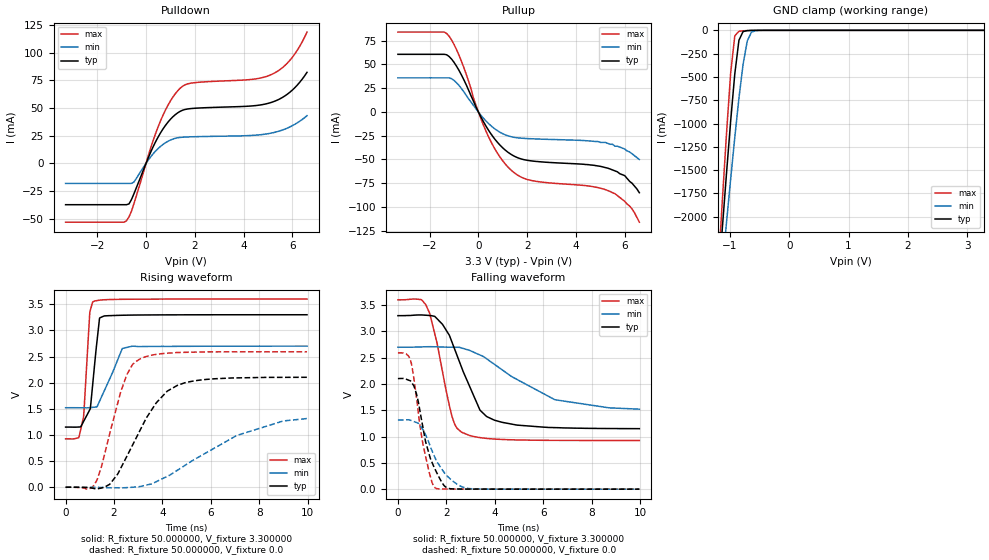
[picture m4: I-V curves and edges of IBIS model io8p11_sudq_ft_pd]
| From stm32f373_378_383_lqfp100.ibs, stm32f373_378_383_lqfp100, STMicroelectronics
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|   Model io8p11_sudq_ft_pd
[Model]  io8p11_sudq_ft_pd
Model_type I/O
Polarity   Non-Inverting
Enable   Active-Low
Vinl =   0.990000V
Vinh =   2.310000V
Vmeas =  1.650000V
Cref =   30.000000pF
Rref =   100.000000M
Vref =   0.0V
C_comp   1.970900pF   1.892300pF   2.063200pF
[Temperature Range]   25.000000   0.125000k   -40.000000
[Pullup Reference]   3.300000V   2.700000V   3.600000V
[Pulldown Reference]   0.0V   0.0V   0.0V
[POWER Clamp Reference]   3.300000V   2.700000V   3.600000V
[GND Clamp Reference]   0.0V   0.0V   0.0V
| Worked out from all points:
|   slope of the pulldown table from 0 to 0.495 V, typ, clamps not added: 20.9 ohm
|   slope of the pullup table from 0 to 0.495 V, typ, clamps not added: 22.2 ohm
|   GND clamp passes 1 mA (typ) near -0.64 V on its own axis
|   rising waveform, R_fixture 50.000000, V_fixture 3.300000: 20-80 % time 277ps typ, 663ps min, 203ps max; typ from 1.15 V to 3.3 V
|   rising waveform, R_fixture 50.000000, V_fixture 0.0: 20-80 % time 1.54ns typ, 3.09ns min, 916ps max; typ from 0 V to 2.1 V
|   falling waveform, R_fixture 50.000000, V_fixture 3.300000: 20-80 % time 1.14ns typ, 2.54ns min, 732ps max; typ from 3.3 V to 1.15 V
|   falling waveform, R_fixture 50.000000, V_fixture 0.0: 20-80 % time 659ps typ, 874ps min, 527ps max; typ from 2.1 V to 0 V
[Pulldown]
|Voltage   I(typ)   I(min)   I(max)
-3.3V     -37.45mA   -18.2mA    -53.24mA
-800mV    -37.45mA   -18.2mA    -51.9mA
-700mV    -36.7mA    -18.2mA    -48.48mA
-500mV    -27.71mA   -17.01mA   -36.66mA
200mV     10.57mA    6.084mA    14.57mA
500mV     23.91mA    13.38mA    33.24mA
900mV     37.17mA    19.88mA    52.48mA
1.3V      45.55mA    23.01mA    65.5mA
1.8V      49.29mA    23.83mA    72.18mA
5.1V      54.68mA    27.07mA    79.72mA
5.9V      64.2mA     32.82mA    93.01mA
6.6V      82.13mA    42.97mA    118.5mA
[Pullup]
|Voltage   I(typ)   I(min)   I(max)
-3.3V     60.68mA    35.92mA    84.08mA
-1.4V     60.68mA    35.92mA    84.08mA
-1.2V     58.37mA    35.92mA    79.66mA
-700mV    39.18mA    24.86mA    53.69mA
0V        0A         0A         0A
400mV     -18.61mA   -11.78mA   -25.23mA
900mV     -35.28mA   -21.55mA   -48mA
1.5V      -46.91mA   -26.86mA   -64.58mA
2.2V      -51.57mA   -28.22mA   -72.25mA
5.3V      -59.1mA    -33mA      -82.6mA
6.2V      -73mA      -42mA      -99mA
6.6V      -85mA      -50mA      -116mA
[GND_clamp]
|Voltage   I(typ)   I(min)   I(max)
-3.3V     -9.525A    -9.501A    -9.513A
-1.2V     -2.719A    -3.023A    -2.568A
-1.13V    -2.122A    -2.541A    -1.826A
-1.06V    -1.537A    -2.065A    -1.111A
-990mV    -975.7mA   -1.599A    -462mA
-920mV    -467.5mA   -1.149A    -59.02mA
-850mV    -106.6mA   -727.3mA   -10.13mA
-780mV    -13.08mA   -365.4mA   -5.271mA
-710mV    -3.06mA    -114.8mA   -2.651mA
-640mV    -957.2uA   -20.17mA   -921.6uA
-570mV    -212.9uA   -3.969mA   -172uA
3.28V     83.81uA    63.75uA    93.54uA
[POWER_clamp]
|Voltage   I(typ)   I(min)   I(max)
-3.28V    0A         0A         0A
0V        0A         0A         0A
[Ramp]
| variable   typ   min   max
dV/dt_r  1.26120/1.54122n   0.74130/3.11733n   1.55376/0.91453n
dV/dt_f  1.28796/1.14240n   0.68838/2.56706n   1.60431/0.73092n
R_load = 50.000000
[Rising Waveform]
R_fixture= 50.000000
V_fixture= 3.300000
V_fixture_min= 2.700000
V_fixture_max= 3.600000
|time   V(typ)   V(min)   V(max)
0s        1.15V      1.521V     925.1mV
540.5ps   1.152V     1.52V      945.8mV
740.7ps   1.256V     1.519V     1.344V
1.001ns   1.484V     1.523V     3.353V
1.121ns   1.976V     1.528V     3.546V
1.401ns   3.231V     1.644V     3.577V
1.602ns   3.276V     1.848V     3.585V
2.342ns   3.289V     2.654V     3.594V
2.763ns   3.292V     2.698V     3.595V
9.97ns    3.299V     2.699V     3.599V
[Rising Waveform]
R_fixture= 50.000000
V_fixture= 0.0
V_fixture_min= 0.0
V_fixture_max= 0.0
|time   V(typ)   V(min)   V(max)
0s        -11.46uV   -27.3uV    -6.454uV
1.181ns   -24.48mV   -1.038mV   43.68mV
1.481ns   -14.37mV   -4.325mV   396.7mV
1.822ns   56.8mV     -9.542mV   1.023V
2.523ns   585.5mV    -6.904mV   2.147V
3.043ns   1.06V      10.75mV    2.445V
3.744ns   1.614V     106.7mV    2.541V
4.905ns   1.995V     410.6mV    2.58V
7.067ns   2.091V     989.9mV    2.59V
9.97ns    2.103V     1.315V     2.59V
[Falling Waveform]
R_fixture= 50.000000
V_fixture= 3.300000
V_fixture_min= 2.700000
V_fixture_max= 3.600000
|time   V(typ)   V(min)   V(max)
0s        3.299V     2.699V     3.599V
961ps     3.312V     2.704V     3.603V
1.161ns   3.307V     2.707V     3.494V
1.622ns   3.237V     2.705V     2.765V
2.222ns   2.807V     2.699V     1.402V
2.623ns   2.323V     2.685V     1.084V
3.383ns   1.508V     2.551V     980.4mV
3.984ns   1.312V     2.373V     953mV
6.486ns   1.17V      1.7V       927.7mV
9.97ns    1.15V      1.521V     925.1mV
[Falling Waveform]
R_fixture= 50.000000
V_fixture= 0.0
V_fixture_min= 0.0
V_fixture_max= 0.0
|time   V(typ)   V(min)   V(max)
0s        2.103V     1.315V     2.59V
340.3ps   2.09V      1.318V     2.571V
560.6ps   2.032V     1.302V     2.382V
760.8ps   1.82V      1.268V     1.76V
1.021ns   1.202V     1.14V      884.6mV
1.401ns   516mV      737mV      137.2mV
1.542ns   370.9mV    588.4mV    24.49mV
2.002ns   31.88mV    262.8mV    2.396mV
2.863ns   1.735mV    16.01mV    907.3uV
9.97ns    -11.46uV   -27.3uV    -6.454uV
